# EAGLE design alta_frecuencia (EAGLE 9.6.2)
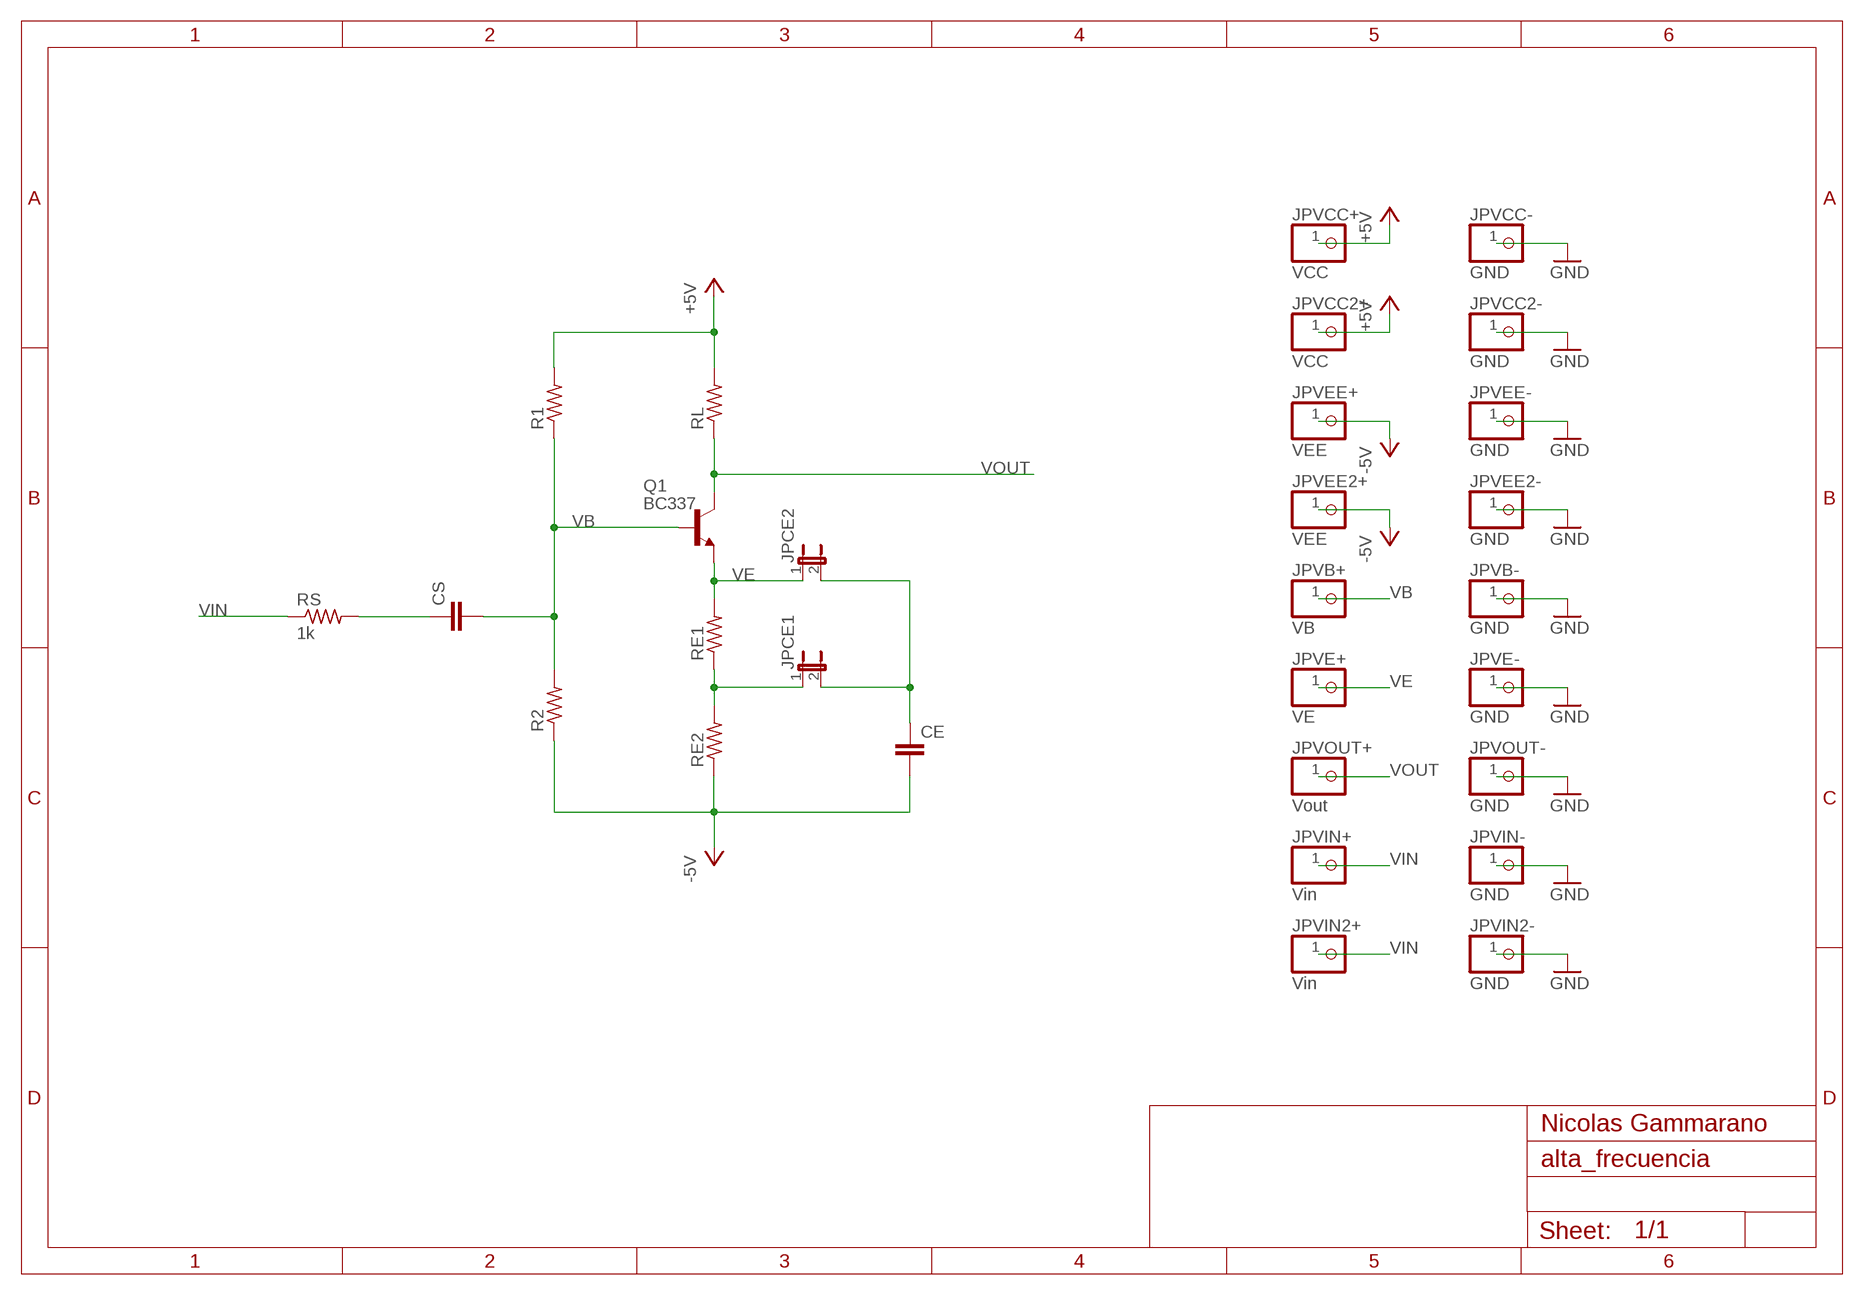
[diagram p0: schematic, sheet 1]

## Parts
CE  C-EU050-035X075  [C050-035X075]
CS  C-EU050-035X075  [C050-035X075]
JPCE1  JP1E  [JP1]
JPCE2  JP1E  [JP1]
JPVB+  VB  PINHD-1X1  [1X01]
JPVB-  GND  PINHD-1X1  [1X01]
JPVCC2+  VCC  PINHD-1X1  [1X01]
JPVCC2-  GND  PINHD-1X1  [1X01]
JPVCC+  VCC  PINHD-1X1  [1X01]
JPVCC-  GND  PINHD-1X1  [1X01]
JPVE+  VE  PINHD-1X1  [1X01]
JPVE-  GND  PINHD-1X1  [1X01]
JPVEE2+  VEE  PINHD-1X1  [1X01]
JPVEE2-  GND  PINHD-1X1  [1X01]
JPVEE+  VEE  PINHD-1X1  [1X01]
JPVEE-  GND  PINHD-1X1  [1X01]
JPVIN2+  Vin  PINHD-1X1  [1X01]
JPVIN2-  GND  PINHD-1X1  [1X01]
JPVIN+  Vin  PINHD-1X1  [1X01]
JPVIN-  GND  PINHD-1X1  [1X01]
JPVOUT+  Vout  PINHD-1X1  [1X01]
JPVOUT-  GND  PINHD-1X1  [1X01]
Q1  BC337  [TO92]
R1  R-US_0207/10  [0207/10]
R2  R-US_0207/10  [0207/10]
RE1  R-US_0207/10  [0207/10]
RE2  R-US_0207/10  [0207/10]
RL  R-US_0207/10  [0207/10]
RS  1k  R-US_0207/10  [0207/10]

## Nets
+5V: JPVCC2+.1 JPVCC+.1 R1.2 RL.2
-5V: CE.2 JPVEE2+.1 JPVEE+.1 R2.1 RE2.1
GND: JPVB-.1 JPVCC2-.1 JPVCC-.1 JPVE-.1 JPVEE2-.1 JPVEE-.1 JPVIN2-.1 JPVIN-.1 JPVOUT-.1
N$3: CS.1 RS.2
N$8: JPCE1.1 RE1.1 RE2.2
N$9: CE.1 JPCE1.2 JPCE2.2
VB: CS.2 JPVB+.1 Q1.2(B) R1.1 R2.2
VE: JPCE2.1 JPVE+.1 Q1.1(E) RE1.2
VIN: JPVIN2+.1 JPVIN+.1 RS.1
VOUT: JPVOUT+.1 Q1.3(C) RL.1

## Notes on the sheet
- Nicolas Gammarano

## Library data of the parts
CE CS = rcl:C-EU: CAPACITOR, European symbol; SPICEPREFIX: C
JPCE1 JPCE2 = jumper:JP1E: JUMPER
JPVB+ JPVB- JPVCC2+ JPVCC2- JPVCC+ JPVCC- JPVE+ JPVE- JPVEE2+ JPVEE2- JPVEE+ JPVEE- JPVIN2+ JPVIN2- JPVIN+ JPVIN- JPVOUT+ JPVOUT- = pinhead:PINHD-1X1: PIN HEADER
Q1 = transistor:BC337: NPN TRANSISTOR
R1 R2 RE1 RE2 RL RS = rcl:R-US_: RESISTOR, American symbol; SPICEPREFIX: R

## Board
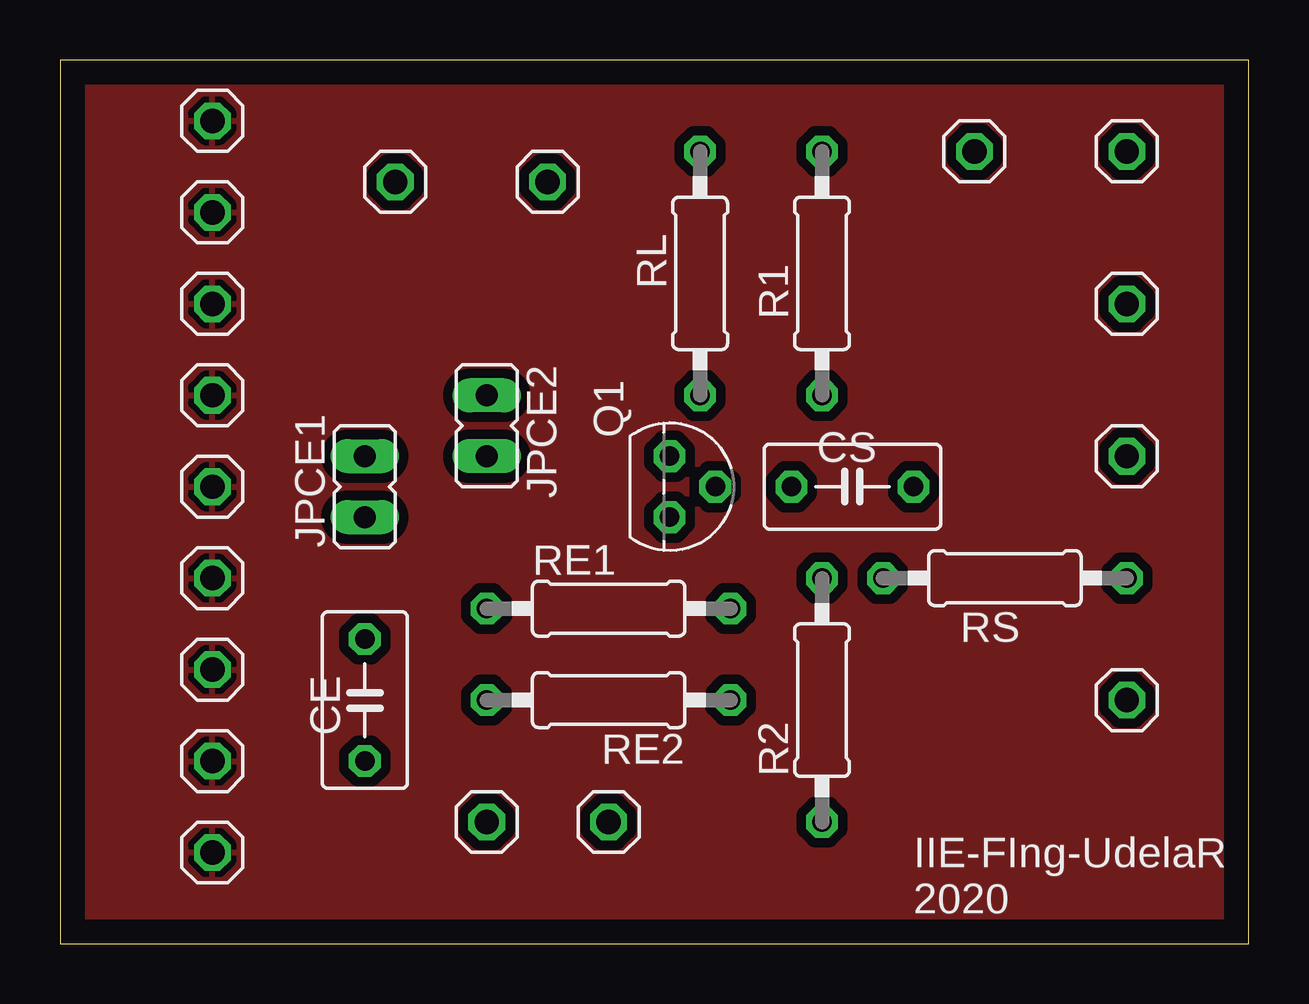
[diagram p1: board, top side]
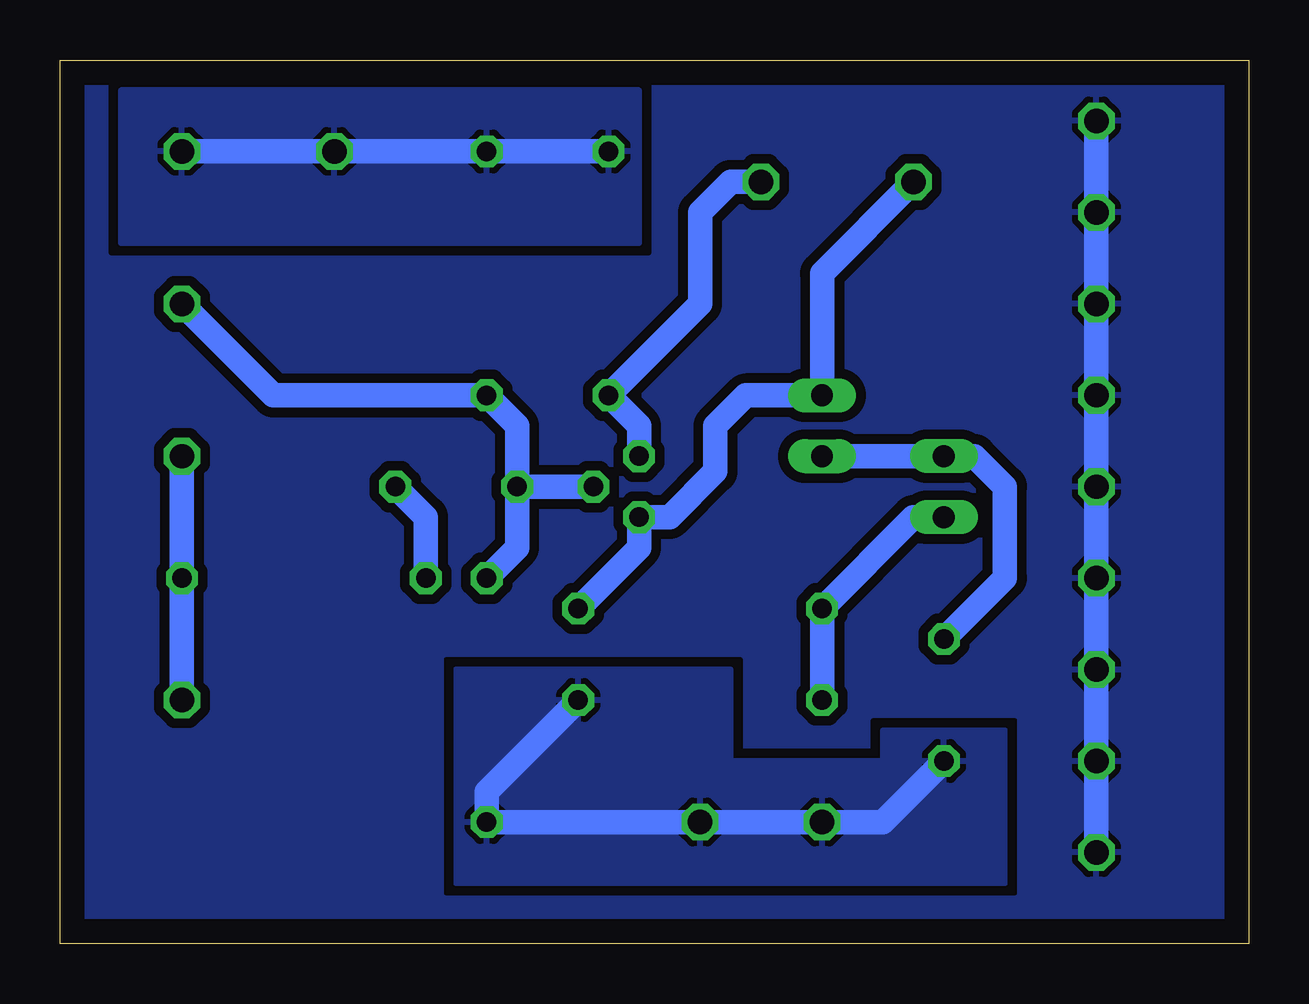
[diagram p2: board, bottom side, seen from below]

Size 49.53 x 36.83 mm. Coordinates in mm from the lower left corner, seen from the top.
Outline: 0,0 49.53,0 49.53,36.83 0,36.83 0,0
Copper layers (1*16): Top 0.035mm / dielectric 1.5mm / Bottom 0.035mm
Design rules "default": minimum track width 6mil, minimum drill 0.35mm, track to track 6mil, track to pad 6mil, pad to pad 6mil, via to via 6mil, smd to smd 6mil, copper to edge 40mil, drill to drill 6mil, minimum pad ring 10mil, minimum via ring 8mil, stop-mask expansion 4mil, vias tented up to drill 0mil, thermal gap 10mil

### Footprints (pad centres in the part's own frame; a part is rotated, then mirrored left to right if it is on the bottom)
C050-035X075 = drill 0.813 octagon: 1 -2.54,0; 2 2.54,0
JP1 = drill 0.914 long: 1 0,-1.27; 2 0,1.27
1X01 = drill 1.016 octagon: 1 0,0
TO92 = drill 0.813 octagon: 1 1.27,0; 2 0,1.905; 3 -1.27,0
0207/10 = drill 0.813 octagon: 1 -5.08,0; 2 5.08,0

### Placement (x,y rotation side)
CE  12.7,10.16 270 top
CS  33.02,19.05 180 top
JPCE1  12.7,19.05 0 top
JPCE2  17.78,21.59 180 top
JPVB+  44.45,26.67 180 top
JPVB-  6.35,19.05 180 top
JPVCC2+  44.45,33.02 0 top
JPVCC2-  6.35,7.62 0 top
JPVCC+  38.1,33.02 180 top
JPVCC-  6.35,11.43 180 top
JPVE+  13.97,31.75 180 top
JPVE-  6.35,26.67 180 top
JPVEE2+  22.86,5.08 0 top
JPVEE2-  6.35,3.81 0 top
JPVEE+  17.78,5.08 180 top
JPVEE-  6.35,15.24 180 top
JPVIN2+  44.45,10.16 180 top
JPVIN2-  6.35,34.29 180 top
JPVIN+  44.45,20.32 180 top
JPVIN-  6.35,22.86 180 top
JPVOUT+  20.32,31.75 180 top
JPVOUT-  6.35,30.48 180 top
Q1  25.4,19.05 270 top
R1  31.75,27.94 90 top
R2  31.75,10.16 90 top
RE1  22.86,13.97 0 top
RE2  22.86,10.16 180 top
RL  26.67,27.94 90 top
RS  39.37,15.24 180 top

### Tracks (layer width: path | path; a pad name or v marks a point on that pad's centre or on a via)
+5V
  Bottom 1.016: JPVCC2+.1 JPVCC+.1 R1.2 RL.2
  pour Bottom (isolate 0.406): 25.4,35.56 46.99,35.56 46.99,29.21 25.4,29.21
-5V
  Bottom 1.016: CE.2 15.24,5.08 JPVEE+.1 JPVEE2+.1 R2.1 31.75,6.35 RE2.1
  pour Bottom (isolate 0.406): 10.16,8.89 15.24,8.89 15.24,7.62 21.59,7.62 21.59,11.43 33.02,11.43 33.02,2.54 10.16,2.54
GND
  Bottom 1.016: JPVIN2-.1 JPVOUT-.1 JPVE-.1 JPVIN-.1 JPVB-.1 JPVEE-.1 JPVCC-.1 JPVCC2-.1 JPVEE2-.1
  pour Bottom (isolate 0.406, rank 2): 0,0 0,36.83 49.53,36.83 49.53,0
  pour Top (isolate 0.406): 0,0 49.53,0 49.53,36.83 0,36.83
N$3
  Bottom 1.016: CS.1 34.29,17.78 RS.2
N$8
  Bottom 1.016: JPCE1.1 13.97,17.78 RE1.1 RE2.2
N$9
  Bottom 1.016: CE.1 10.16,15.24 10.16,19.05 11.43,20.32 JPCE1.2 JPCE2.2
VB
  Bottom 1.016: CS.2 30.48,21.59 R1.1 40.64,22.86 JPVB+.1 | R2.2 30.48,16.51 CS.2 | CS.2 Q1.2
VE
  Bottom 1.016: RE1.2 25.4,16.51 Q1.1 24.13,17.78 22.23,19.68 22.23,21.59 20.95,22.86 JPCE2.1 17.78,27.94 JPVE+.1
VIN
  Bottom 1.016: JPVIN+.1 RS.1 JPVIN2+.1
VOUT
  Bottom 1.016: Q1.3 25.4,21.59 RL.1 22.86,26.67 22.86,30.48 21.59,31.75 JPVOUT+.1

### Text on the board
tNames: IIE-FIng-UdelaR / 2020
